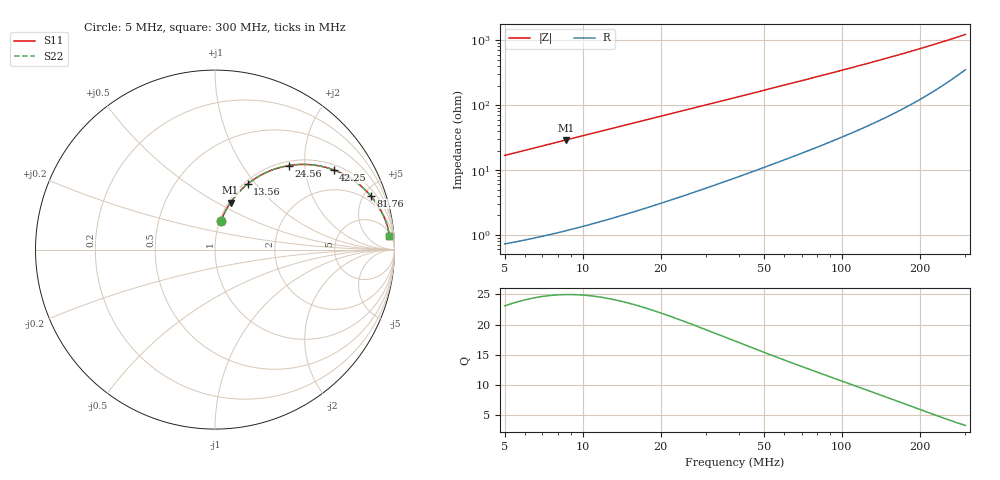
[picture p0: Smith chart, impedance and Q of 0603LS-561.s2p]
# MHz S MA R 50
!Freq  MagS11  AngS11  MagS21  AngS21  MagS12  AngS12  MagS22  AngS22
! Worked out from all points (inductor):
!   801 points, 5 MHz to 300 MHz, reference 50 ohm
!   read as one part in series: L = 535 nH near 5.103 MHz
!   highest Q = 25 at 8.646 MHz (marker M1), where L = 535 nH
!   S11 on the Smith chart (normalised r, x): 5 MHz: 1.01, +0.34; 13.56 MHz: 1.04, +0.91; 24.56 MHz: 1.08, +1.65; 42.25 MHz: 1.17, +2.84; 81.76 MHz: 1.46, +5.56; 300 MHz: 8, +23
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5  0.1647 78.1  0.9793 -9.5  0.9793 -9.5  0.1647 78.1
6.728  0.2187 75.0  0.9669 -12.6  0.9669 -12.6  0.2187 75.0
8.645652  0.2762 71.7  0.9501 -16.0  0.9501 -16.0  0.2762 71.7
10.94061  0.3408 67.8  0.9265 -19.9  0.9265 -19.9  0.3408 67.8
13.56421  0.4086 63.5  0.8959 -24.1  0.8959 -24.1  0.4086 63.5
15.89636  0.4632 60.0  0.8666 -27.6  0.8666 -27.6  0.4632 60.0
18.53439  0.5187 56.2  0.8322 -31.2  0.8322 -31.2  0.5187 56.2
21.39014  0.5715 52.5  0.7944 -34.8  0.7944 -34.8  0.5715 52.5
24.55988  0.6223 48.8  0.7531 -38.4  0.7531 -38.4  0.6223 48.8
28.63565  0.6768 44.5  0.7022 -42.5  0.7022 -42.5  0.6768 44.5
33.21735  0.7262 40.4  0.6492 -46.5  0.6492 -46.5  0.7262 40.4
42.25045  0.7964 33.9  0.5589 -52.7  0.5589 -52.7  0.7964 33.9
48.01739  0.828 30.6  0.5106 -55.7  0.5106 -55.7  0.828 30.6
54.29291  0.8544 27.7  0.4653 -58.5  0.4653 -58.5  0.8544 27.7
66.62706  0.8904 23.1  0.3938 -62.6  0.3938 -62.6  0.8904 23.1
81.76327  0.9175 19.1  0.3289 -66.1  0.3289 -66.1  0.9175 19.1
103.467  0.9399 15.2  0.2636 -69.3  0.2636 -69.3  0.9399 15.2
126.3243  0.9531 12.4  0.2162 -71.3  0.2162 -71.3  0.9531 12.4
152.6604  0.962 10.1  0.1774 -72.6  0.1774 -72.6  0.962 10.1
202.2899  0.9702 7.3  0.1296 -73.1  0.1296 -73.1  0.9702 7.3
252.0866  0.9734 5.6  0.09938 -71.7  0.09938 -71.7  0.9734 5.6
300  0.9743 4.4  0.0795 -69.0  0.0795 -69.0  0.9743 4.4
